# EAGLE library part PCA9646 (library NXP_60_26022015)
The PCA9646 is a monolithic CMOS integrated circuit for 2-wire bus buffering and switching in applications including I2C-bus, SMBus, PMBus, and other systems based on similar principles. AAL Eindhoven MK
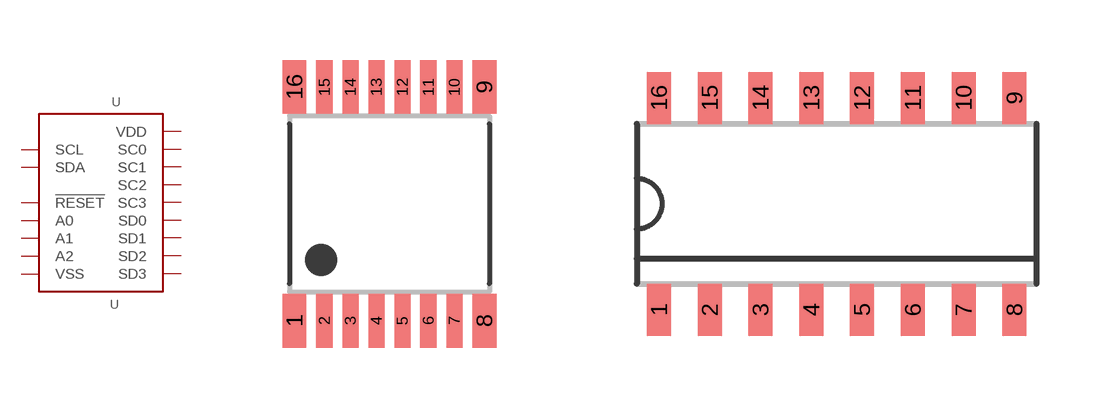
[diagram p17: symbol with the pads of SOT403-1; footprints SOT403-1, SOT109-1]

Designator prefix U

## PCA9646PW  [SOT403-1]
1  A0  in
2  A1  in
3  !RESET  in
4  SD0
5  SC0
6  SD1
7  SC1
8  VSS  pwr
9  SD2
10  SC2
11  SD3
12  SC3
13  A2  in
14  SCL
15  SDA
16  VDD  pwr

## PCA9646P  [SOT109-1]
Pads as for SOT403-1

## Footprint SOT403-1 (pad centres in mm)
SOT403-1 TSSOP16: plastic thin shrink small outline package; 16 leads; body width 4.4 mm JEDEC: MO-153 IEC: ---
smd 0.6 x 1.35: 1 -2.375,-2.925; 8 2.375,-2.925; 9 2.375,2.925; 16 -2.375,2.925
smd 0.4 x 1.35: 2 -1.625,-2.925; 3 -0.975,-2.925; 4 -0.325,-2.925; 5 0.325,-2.925; 6 0.975,-2.925; 7 1.625,-2.925; 10 1.625,2.925; 11 0.975,2.925; 12 0.325,2.925; 13 -0.325,2.925; 14 -0.975,2.925; 15 -1.625,2.925

## Footprint SOT109-1 (pad centres in mm)
SOT109-1 SO16: plastic small outline package; 16 leads; body width 3.9 mm JEDEC: MS-012 IEC: 076E07
smd 0.6 x 1.3: 1 -4.445,-2.65; 2 -3.175,-2.65; 3 -1.905,-2.65; 4 -0.635,-2.65; 5 0.635,-2.65; 6 1.905,-2.65; 7 3.175,-2.65; 8 4.445,-2.65; 9 4.445,2.65; 10 3.175,2.65; 11 1.905,2.65; 12 0.635,2.65; 13 -0.635,2.65; 14 -1.905,2.65; 15 -3.175,2.65; 16 -4.445,2.65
